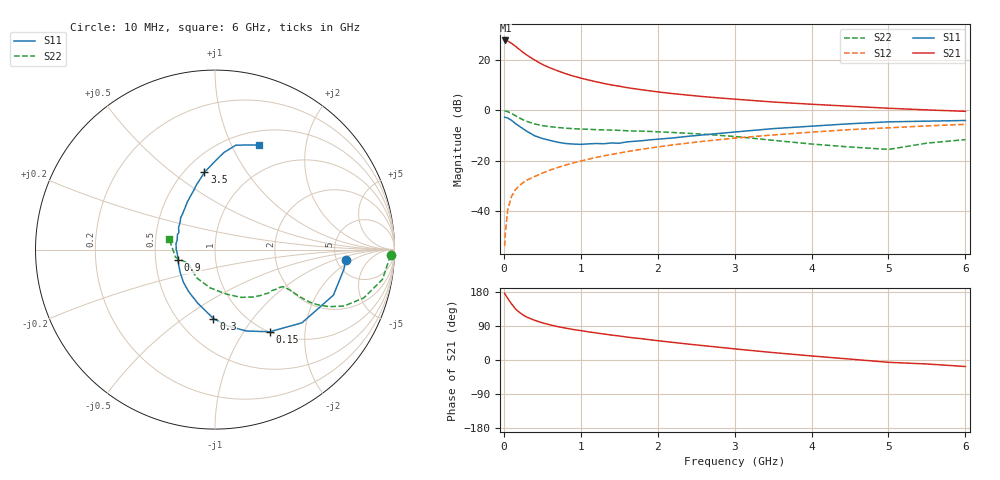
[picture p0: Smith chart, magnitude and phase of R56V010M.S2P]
! SIEMENS Small Signal Semiconductors
! BFR183
! Si NPN RF Bipolar Junction Transistor in SOT23
! VCE = 6 V  IC = 10 mA
! Common Emitter S-Parameters:  May  1996
# GHz  S  MA  R  50
!  f  S11  S21  S12  S22
! GHz  MAG  ANG  MAG  ANG  MAG  ANG  MAG  ANG
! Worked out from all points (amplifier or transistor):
!   36 points, 10 MHz to 6 GHz, reference 50 ohm
!   highest |S21| = 27.8 dB at 20 MHz (marker M1)
!   |S21| within 3 dB of that: start of sweep to 179.3 MHz
!   unconditionally stable (mu >= 1): 799.5 MHz to 2.562 GHz
!   at 250 MHz: K = 0.61, MSG = 25.9 dB, |S12| = -28.7 dB
!   at 1.4 GHz: K = 1.05, MAG = 12.5 dB, |S12| = -17.5 dB
!   at 6 GHz: K = 0.89, MSG = 2.6 dB, |S12| = -5.5 dB
!   lowest NFmin = 1.30 dB at 450 MHz
!   S11 on the Smith chart (normalised r, x): 10 MHz: 6.08, -1.50; 150 MHz: 1.01, -1.32; 300 MHz: 0.73, -0.66; 900 MHz: 0.65, -0.08; 3.5 GHz: 0.62, +0.66; 6 GHz: 0.66, +1.28
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0.01  0.7319 -4.5  24.52 176.2  0.002 84.3  0.9787 -1.9
0.02  0.7264 -8.7  24.59 172.5  0.0037 84.0  0.9682 -4.1
0.05  0.707 -21.0  23.96 162.7  0.0105 79.7  0.9476 -10.1
0.1  0.6335 -40.1  21.56 148.1  0.0195 73.4  0.8712 -18.0
0.15  0.5496 -56.4  18.91 135.1  0.0264 66.8  0.7853 -23.6
0.2  0.4862 -68.9  16.42 126.2  0.0319 64.5  0.7104 -26.6
0.25  0.4306 -80.8  14.25 118.8  0.0366 62.8  0.6516 -28.2
0.3  0.3843 -91.3  12.58 113.0  0.0412 62.6  0.605 -29.0
0.4  0.3135 -107.9  10.03 104.8  0.0485 63.3  0.5391 -29.1
0.5  0.2768 -121.9  8.222 98.0  0.0565 63.7  0.4992 -28.7
0.6  0.2533 -133.8  7.013 92.8  0.065 64.5  0.4752 -28.4
0.7  0.2335 -145.9  6.117 88.1  0.0732 65.2  0.4578 -28.4
0.9  0.2145 -164.3  4.828 80.6  0.0904 65.6  0.4334 -28.6
1.1  0.2162 179.4  4.027 74.4  0.1074 65.3  0.4208 -30.0
1.3  0.2176 165.5  3.437 68.6  0.125 64.5  0.4099 -31.6
1.6  0.2371 149.0  2.841 60.5  0.1515 62.8  0.394 -35.1
2.2  0.2839 126.4  2.153 46.5  0.2065 58.2  0.3641 -44.3
2.8  0.3486 110.1  1.77 33.6  0.2624 52.1  0.3188 -56.1
3.5  0.4343 97.8  1.47 19.6  0.3251 43.6  0.2545 -76.2
4.5  0.5427 84.8  1.209 2.4  0.4156 31.6  0.1872 -123.5
5.5  0.6111 72.6  1.023 -10.5  0.4926 20.0  0.2237 -168.9
6  0.6307 67.3  0.96 -17.2  0.529 12.3  0.2626 167.0
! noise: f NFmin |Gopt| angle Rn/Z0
0.45  1.3  0.15  45  0.18
0.9  1.4  0.2  125  0.19
1.8  2.1  0.34  -170  0.14
